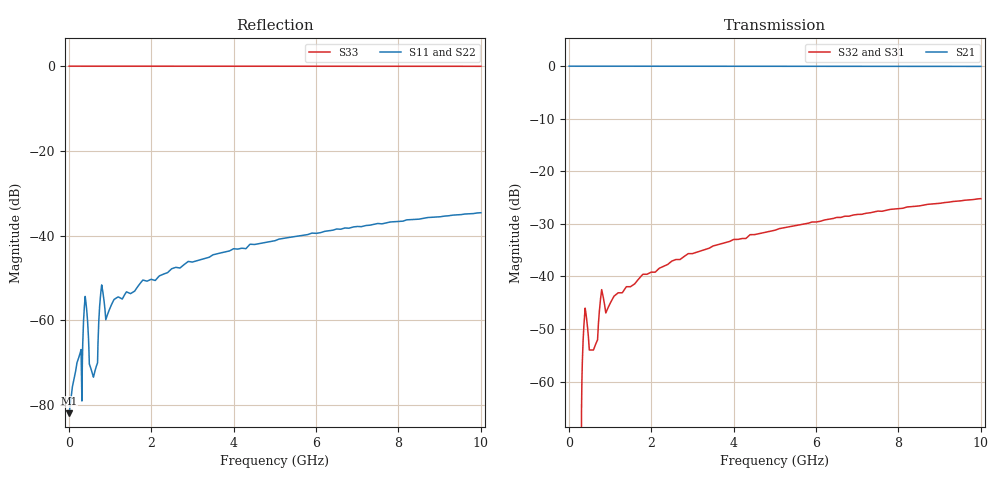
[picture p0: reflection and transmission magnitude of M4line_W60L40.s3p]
! Created Fri Sep 09 14:08:53 2011
# ghz S ma R 50
! 3 Port Network Data from SP1.SP block
! freq  magS11  angS11  magS12  angS12  magS13  angS13
!  magS21  angS21
!  magS22  angS22  magS23  angS23
!  magS31  angS31  magS32  angS32
!  magS33  angS33
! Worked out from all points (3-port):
!   1000 points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, 10 MHz to 10 GHz, reference 50 ohm
!   strongest paths, dB at 10 MHz, 2.51 GHz, 5.01 GHz, 7.51 GHz, 10 GHz:
!     S21: 0.0, 0.0, 0.0, 0.0, 0.0
!     S32: -, -37.0, -31.2, -27.6, -25.2
!     S31: -, -37.0, -31.2, -27.6, -25.2
!   lowest |S11| = -81.9 dB at 10 MHz (marker M1), VSWR 1.00, Z = 50 + j0.00156 ohm
!   |S11| at or under -10 dB: start of sweep to end of sweep
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0.01  8.026e-05 11.2  0.9999 -0.0  0 0.0
      0.9999 -0.0  8.026e-05 11.2  0 0.0
      0 0.0  0 0.0  1 0.0
0.25  0.0003728 74.8  0.9999 -0.0  0 0.0
      0.9999 -0.0  0.0003728 74.8  0 0.0
      0 0.0  0 0.0  1 0.0
0.3  0.0004534 76.8  0.9999 -0.0  0 0.0
     0.9999 -0.0  0.0004534 76.8  0 0.0
     0 0.0  0 0.0  1 0.0
0.39  0.00169 -86.5  0.9999 -0.2  0.0045 89.6
      0.9999 -0.2  0.00169 -86.5  0.0045 89.6
      0.0045 89.6  0.0045 89.6  1 -0.5
0.61  0.0002246 -42.5  0.9998 -0.1  0.00205 89.8
      0.9998 -0.1  0.0002246 -42.5  0.00205 89.8
      0.00205 89.8  0.00205 89.8  1 -0.2
0.81  0.002467 -85.7  0.9997 -0.3  0.0072 89.4
      0.9997 -0.3  0.002467 -85.7  0.0072 89.4
      0.0072 89.4  0.0072 89.4  0.9999 -0.8
0.94  0.00117 -77.7  0.9997 -0.2  0.0049 89.6
      0.9997 -0.2  0.00117 -77.7  0.0049 89.6
      0.0049 89.6  0.0049 89.6  1 -0.6
1.8  0.002997 -80.1  0.9993 -0.4  0.0105 89.1
     0.9993 -0.4  0.002997 -80.1  0.0105 89.1
     0.0105 89.1  0.0105 89.1  0.9999 -1.2
5.01  0.00874 -83.1  0.9979 -1.1  0.02757 87.4
      0.9979 -1.1  0.00874 -83.1  0.02757 87.4
      0.02757 87.4  0.02757 87.4  0.999 -3.2
10  0.01866 -88.0  0.9952 -2.1  0.05499 85.0
    0.9952 -2.1  0.01866 -88.0  0.05499 85.0
    0.05499 85.0  0.05499 85.0  0.9965 -6.3
